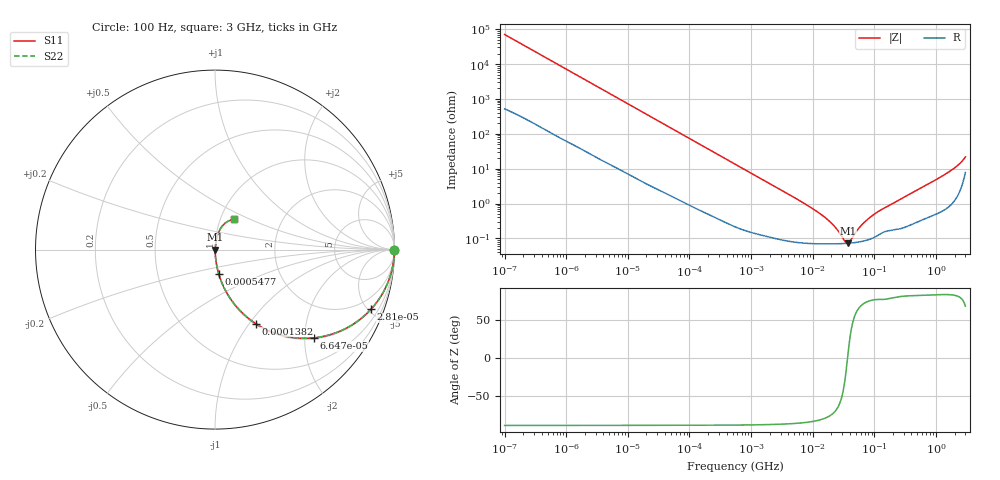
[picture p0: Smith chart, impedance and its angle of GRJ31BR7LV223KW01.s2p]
!Murata Part Number: GRJ31BR7LV223KW01
!These Parameters are Measured in Series Mode Connection
!Data Generated on Jun 19, 2026
!  o--ll--o
!Port1  Port2
!  o------o
!Operation Temp=25[degC], DC Bias Voltage=0[V]
!Freq. Start=100[Hz] Stop=3[GHz] 401[Steps]
# Hz S RI R 50
!Freq.(Hz) S11(Real) S11(Imag) S21(Real) S21(Imag) S12(Real) S12(Imag) S22(Real) S22(Imag)
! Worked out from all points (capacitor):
!   401 points, 100 Hz to 3 GHz, reference 50 ohm
!   read as one part in series: C = 22.4 nF near 109 Hz
!   lowest |Z| = 72.7 mohm at 37.19 MHz (marker M1)
!   series resonance near 36.74 MHz, so ESL is about 840 pH
!   S11 on the Smith chart (normalised r, x): 100 Hz: open; 28.1 kHz: 1.05, -5.21; 66.47 kHz: 1.03, -2.22; 138.2 kHz: 1.01, -1.07; 547.7 kHz: 1.00, -0.27; 3 GHz: 1.16, +0.41
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100  1 -0.00141  1.23e-05 0.00141  1.23e-05 0.00141  1 -0.00141
1788  0.9992 -0.0248  0.000836 0.0248  0.000836 0.0248  0.9992 -0.0248
8421  0.9857 -0.114  0.0143 0.114  0.0143 0.114  0.9857 -0.114
28103  0.8691 -0.3322  0.1309 0.3322  0.1309 0.3322  0.8691 -0.3322
31977  0.8375 -0.3637  0.1625 0.3637  0.1625 0.3637  0.8375 -0.3637
66468  0.5507 -0.4917  0.4493 0.4917  0.4493 0.4917  0.5507 -0.4917
138163  0.226 -0.412  0.774 0.412  0.774 0.412  0.226 -0.412
252400  0.0831 -0.2692  0.9169 0.2692  0.9169 0.2692  0.0831 -0.2692
547723  0.0203 -0.1335  0.9797 0.1335  0.9797 0.1335  0.0203 -0.1335
1677156  0.00317 -0.0447  0.9968 0.0447  0.9968 0.0447  0.00317 -0.0447
9794414  0.000759 -0.00722  0.9992 0.00722  0.9992 0.00722  0.000759 -0.00722
1.950129e7  0.000701 -0.0028  0.9993 0.0028  0.9993 0.0028  0.000701 -0.0028
2.52476e7  0.000702 -0.00159  0.9993 0.00159  0.9993 0.00159  0.000702 -0.00159
3.268714e7  0.000714 -0.000484  0.9993 0.000484  0.9993 0.000484  0.000714 -0.000484
3.71925e7  0.000724 5.19e-05  0.9993 -5.19e-05  0.9993 -5.19e-05  0.000724 5.19e-05
4.0536e7  0.000734 0.000409  0.9993 -0.000409  0.9993 -0.000409  0.000734 0.000409
5.719833e7  0.000797 0.00189  0.9992 -0.00189  0.9992 -0.00189  0.000797 0.00189
7.405258e7  0.000888 0.00314  0.9991 -0.00314  0.9991 -0.00314  0.000888 0.00314
1.090876e8  0.00119 0.00537  0.9988 -0.00537  0.9988 -0.00537  0.00119 0.00537
1.751444e8  0.00174 0.00868  0.9983 -0.00868  0.9983 -0.00868  0.00174 0.00868
1.382454e9  0.011 0.0662  0.989 -0.0662  0.989 -0.0662  0.011 0.0662
3e9  0.1037 0.1684  0.8963 -0.1684  0.8963 -0.1684  0.1037 0.1684
